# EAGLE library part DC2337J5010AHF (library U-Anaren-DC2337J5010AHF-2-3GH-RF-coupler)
Anaren Xinger Series 10dB Directional Coupler
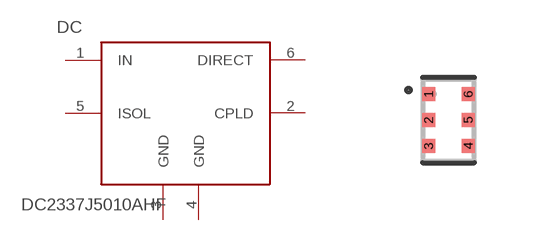
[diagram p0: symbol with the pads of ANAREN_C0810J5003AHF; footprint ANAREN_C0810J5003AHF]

Designator prefix DC

## DC2337J5010AHFDC2337J50 (VALUE: DC2337J5010)  [ANAREN_C0810J5003AHF]
1  IN  in
2  CPLD  out
3  GND
4  GND
5  ISOL  out
6  DIRECT  out

## Footprint ANAREN_C0810J5003AHF (pad centres in mm)
smd 0.33 x 0.35: 1 -0.495,0.65; 2 -0.495,0; 3 -0.495,-0.65; 4 0.495,-0.65; 5 0.495,0; 6 0.495,0.65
